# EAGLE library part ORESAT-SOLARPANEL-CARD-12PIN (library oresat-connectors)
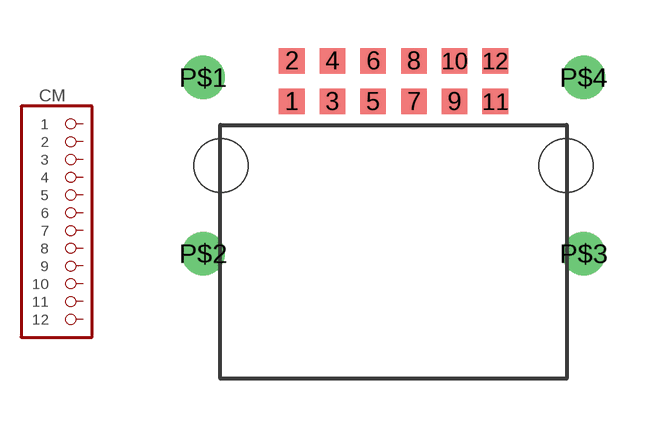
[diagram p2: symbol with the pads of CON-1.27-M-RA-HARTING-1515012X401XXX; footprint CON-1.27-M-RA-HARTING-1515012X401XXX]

Designator prefix CM

## ORESAT-SOLARPANEL-CARD-12PIN  [CON-1.27-M-RA-HARTING-1515012X401XXX]
1  1  pas
2  2  pas
3  3  pas
4  4  pas
5  5  pas
6  6  pas
7  7  pas
8  8  pas
9  9  pas
10  10  pas
11  11  pas
12  12  pas

## Footprint CON-1.27-M-RA-HARTING-1515012X401XXX (pad centres in mm)
smd 0.8 x 0.8: 1 -3.175,2; 2 -3.175,3.27; 3 -1.905,2; 4 -1.905,3.27; 5 -0.635,2; 6 -0.635,3.27; 7 0.635,2; 8 0.635,3.27; 9 1.905,2; 10 1.905,3.27; 11 3.175,2; 12 3.175,3.27
drill 0.6 pad 1.35: P$1 -5.935,2.75; P$2 -5.935,-2.75; P$3 5.935,-2.75; P$4 5.935,2.75
hole 1.68 at 5.385,0
hole 1.68 at -5.385,0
